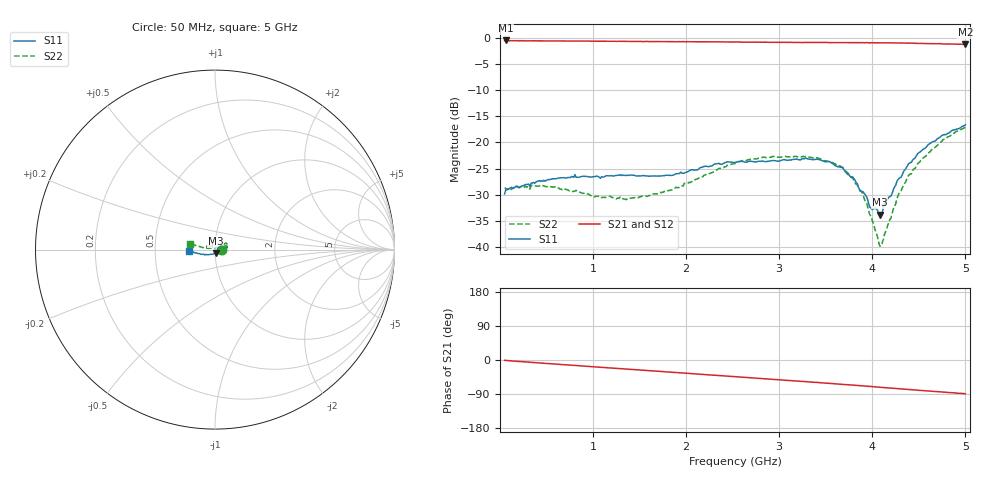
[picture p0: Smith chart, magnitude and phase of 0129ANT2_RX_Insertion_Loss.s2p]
! MASWSS0129 de-embedded Sparameters using port extention method. ANT2 to RX Insertion Loss using 3 volt control
! Board loss is removed and phase length of connector and line length of board are dialed out
! 100pF blocking capacitor
! Sample board 1000013136
#	Hz	S	DB	R	50
!	Freq	S11	S21	S12	S22
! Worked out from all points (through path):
!   401 points, 50 MHz to 5 GHz, reference 50 ohm
!   highest |S21| = -0.49 dB at 62.4 MHz (marker M1); lowest = -1.2 dB at 5 GHz (marker M2)
!   group delay of S21, straight-line fit = 49 ps
!   lowest |S11| = -33.8 dB at 4.08 GHz (marker M3), VSWR 1.04, Z = 50.3 - j2.02 ohm
!   |S11| at or under -10 dB: start of sweep to end of sweep
!   |S22| runs from -39.9 to -17.1 dB; largest |S21 - S12| = 0.0094
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5e7  -29.87 -5.6  -0.54 -0.8  -0.48 -1.2  -28.68 -0.8
6.24e7  -29.04 -6.5  -0.49 -1.1  -0.52 -1.2  -28.80 -0.9
4.46e8  -27.31 6.0  -0.57 -8.2  -0.58 -8.2  -28.25 9.1
8.79e8  -26.51 -4.8  -0.62 -15.7  -0.61 -15.7  -29.70 7.6
1.35e9  -26.36 -6.2  -0.66 -23.9  -0.66 -23.8  -30.95 15.3
1.7e9  -26.47 -0.4  -0.70 -29.7  -0.71 -29.8  -29.84 27.0
2.53e9  -23.82 8.0  -0.79 -44.0  -0.80 -44.1  -24.02 31.2
2.82e9  -23.58 10.9  -0.81 -49.1  -0.84 -49.3  -22.88 29.6
3.35e9  -23.29 12.0  -0.88 -58.5  -0.88 -58.5  -22.91 20.0
3.63e9  -24.65 5.1  -0.91 -63.3  -0.89 -63.4  -24.27 18.2
3.79e9  -26.61 -4.6  -0.91 -66.1  -0.90 -66.4  -26.85 22.9
3.89e9  -29.39 -18.9  -0.92 -68.1  -0.91 -68.2  -29.60 27.8
3.94e9  -30.44 -23.3  -0.89 -69.0  -0.93 -69.1  -31.54 33.2
3.97e9  -32.29 -34.0  -0.91 -69.8  -0.93 -69.8  -33.69 37.4
4.08e9  -33.83 -81.8  -0.93 -71.8  -0.93 -72.0  -39.86 90.4
4.11e9  -33.21 -99.2  -0.93 -72.4  -0.95 -72.4  -39.03 112.9
4.18e9  -30.47 -118.0  -0.93 -73.8  -0.96 -74.0  -35.08 151.8
4.29e9  -26.84 -141.7  -0.97 -75.9  -1.00 -76.1  -29.63 167.7
4.39e9  -24.06 -153.1  -1.00 -77.8  -1.03 -78.1  -26.28 170.7
4.49e9  -22.09 -160.8  -1.05 -79.8  -1.05 -79.9  -24.00 170.3
4.76e9  -18.58 -171.6  -1.16 -84.8  -1.17 -85.0  -19.46 167.6
5e9  -16.64 -177.6  -1.23 -89.3  -1.26 -89.5  -17.06 167.1
